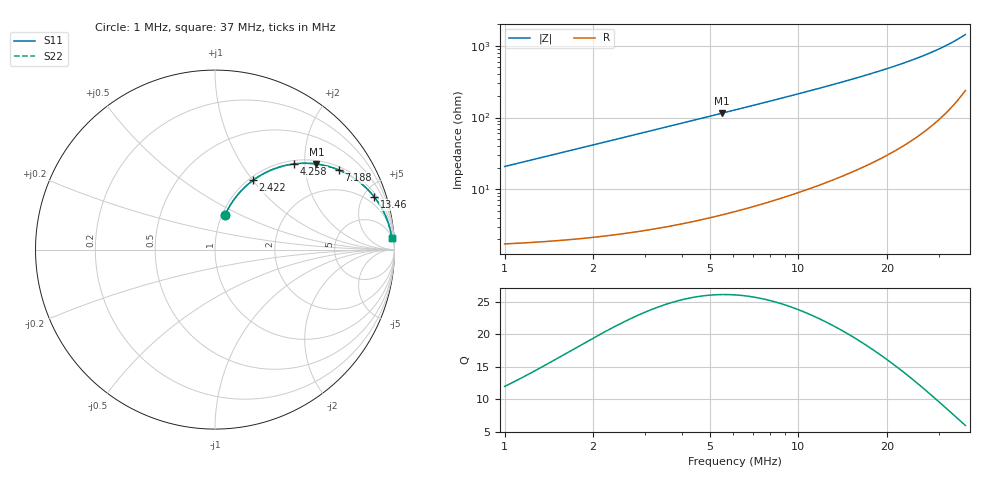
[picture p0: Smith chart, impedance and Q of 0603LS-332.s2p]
# MHz S MA R 50
!Freq  MagS11  AngS11  MagS21  AngS21  MagS12  AngS12  MagS22  AngS22
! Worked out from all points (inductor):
!   801 points, 1 MHz to 37 MHz, reference 50 ohm
!   read as one part in series: L = 3.29 uH near 1.018 MHz
!   highest Q = 26.1 at 5.483 MHz (marker M1), where L = 3.32 uH
!   S11 on the Smith chart (normalised r, x): 1 MHz: 1.03, +0.41; 2.422 MHz: 1.05, +1.00; 4.258 MHz: 1.07, +1.77; 7.188 MHz: 1.12, +3.02; 13.46 MHz: 1.28, +5.93; 37 MHz: 6, +28
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1  0.1999 73.7  0.9633 -11.5  0.9633 -11.5  0.1999 73.7
1.299256  0.2557 71.3  0.9495 -14.8  0.9495 -14.8  0.2557 71.3
1.620866  0.3129 68.4  0.9317 -18.2  0.9317 -18.2  0.3129 68.4
1.994888  0.3753 65.0  0.9078 -22.0  0.9078 -22.0  0.3753 65.0
2.422197  0.4406 61.2  0.8774 -26.1  0.8774 -26.1  0.4406 61.2
2.811239  0.4944 57.9  0.8479 -29.6  0.8479 -29.6  0.4944 57.9
3.248073  0.5486 54.4  0.8136 -33.2  0.8136 -33.2  0.5486 54.4
4.258346  0.6507 47.2  0.7344 -40.6  0.7344 -40.6  0.6507 47.2
5.48296  0.7395 40.2  0.6455 -47.6  0.6455 -47.6  0.7395 40.2
6.249746  0.7805 36.5  0.5959 -51.3  0.5959 -51.3  0.7805 36.5
7.027954  0.8137 33.4  0.5505 -54.4  0.5505 -54.4  0.8137 33.4
7.188366  0.8197 32.8  0.5418 -55.0  0.5418 -55.0  0.8197 32.8
8.38067  0.8568 28.8  0.4826 -58.9  0.4826 -58.9  0.8568 28.8
9.726735  0.8868 25.2  0.4267 -62.4  0.4267 -62.4  0.8868 25.2
11.289  0.9114 21.9  0.3734 -65.6  0.3734 -65.6  0.9114 21.9
13.04318  0.9307 18.9  0.325 -68.4  0.325 -68.4  0.9307 18.9
13.46187  0.9344 18.3  0.3148 -69.0  0.3148 -69.0  0.9344 18.3
15.98066  0.9513 15.2  0.2626 -71.8  0.2626 -71.8  0.9513 15.2
19.05657  0.9642 12.3  0.2141 -74.3  0.2141 -74.3  0.9642 12.3
25.0969  0.9775 8.5  0.1476 -77.0  0.1476 -77.0  0.9775 8.5
31.02786  0.9835 5.9  0.1026 -77.8  0.1026 -77.8  0.9835 5.9
37  0.9864 3.9  0.06858 -76.6  0.06858 -76.6  0.9864 3.9
